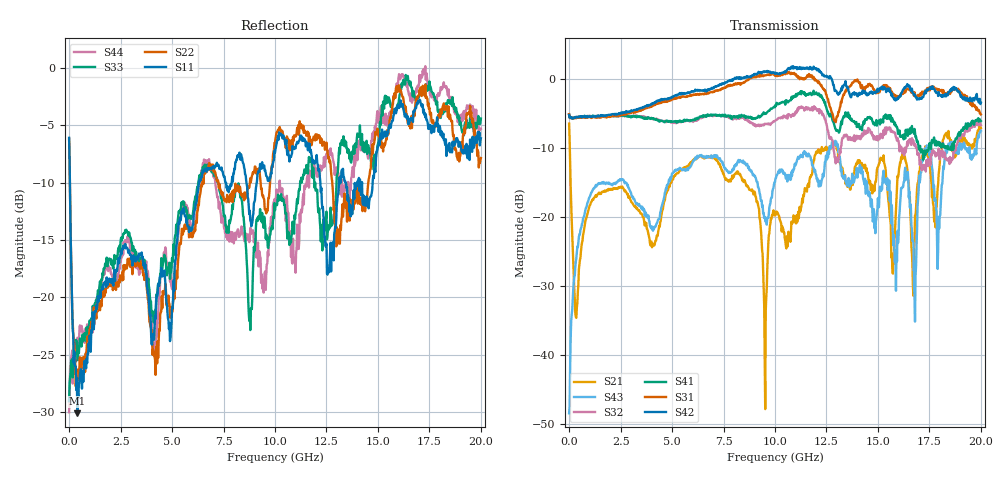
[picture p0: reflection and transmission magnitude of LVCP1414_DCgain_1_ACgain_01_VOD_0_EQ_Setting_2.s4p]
!Agilent Technologies,N5230A,MY46400459,A.07.50.48
!Agilent N5230A: A.07.50.48
!Date: Tuesday, April 17, 2012 18:45:42
!Correction: S11(Full 4 Port(1,2,3,4))
!S12(Full 4 Port(1,2,3,4))
!S13(Full 4 Port(1,2,3,4))
!S14(Full 4 Port(1,2,3,4))
!S21(Full 4 Port(1,2,3,4))
!S22(Full 4 Port(1,2,3,4))
!S23(Full 4 Port(1,2,3,4))
!S24(Full 4 Port(1,2,3,4))
!S31(Full 4 Port(1,2,3,4))
!S32(Full 4 Port(1,2,3,4))
!S33(Full 4 Port(1,2,3,4))
!S34(Full 4 Port(1,2,3,4))
!S41(Full 4 Port(1,2,3,4))
!S42(Full 4 Port(1,2,3,4))
!S43(Full 4 Port(1,2,3,4))
!S44(Full 4 Port(1,2,3,4))
!S4P File: Measurements: <S11,S12,S13,S14>,
!<S21,S22,S23,S24>,
!<S31,S32,S33,S34>,
!<S41,S42,S43,S44>:
# Hz S  dB  R 50
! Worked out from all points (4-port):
!   801 points, 300 kHz to 20 GHz, reference 50 ohm
!   strongest paths, dB at 300 kHz, 5 GHz, 10 GHz, 15 GHz, 20 GHz:
!     S42: -5.3, -2.7, 0.7, -1.6, -3.5
!     S31: -5.2, -3.0, 0.4, -2.1, -5.2
!     S41: -5.2, -6.2, -4.2, -6.3, -6.1
!     S32: -5.2, -6.3, -6.1, -9.0, -6.8
!     S43: -48.4, -13.7, -15.0, -17.3, -7.5
!     S21: -6.5, -14.6, -19.8, -12.8, -7.2
!   lowest |S11| = -30.1 dB at 400.3 MHz (marker M1), VSWR 1.06, Z = 52.9 + j1.36 ohm
!   |S11| at or under -10 dB: 37.38 MHz to 6.309 GHz (6.272 GHz wide, 198 % of centre); 12.2 GHz to 13.11 GHz (907.5 MHz wide, 7.17 % of centre); 13.42 GHz to 14 GHz (575.5 MHz wide, 4.2 % of centre)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
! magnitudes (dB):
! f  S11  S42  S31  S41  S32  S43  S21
! 300 kHz  -6.1  -5.3  -5.2  -5.2  -5.2  -48.4  -6.5
! 400.3 MHz  -30.1  -5.6  -5.6  -5.6  -5.6  -24.3  -32.5
! 10.1 GHz  -6.4  0.8  0.4  -3.6  -5.9  -13.9  -19.4
! 12.75 GHz  -15.3  -0.1  -4.8  -5.5  -8.8  -9.6  -9.9
! 16.78 GHz  -3.8  -2.3  -2.0  -7.3  -9.7  -31.2  -24.0
! 17.4 GHz  -4.7  -1.7  -1.4  -10.4  -11.8  -10.2  -10.1
! 20 GHz  -6.1  -3.5  -5.2  -6.1  -6.8  -7.5  -7.2
